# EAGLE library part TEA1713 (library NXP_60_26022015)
Resonant power supply control IC with PFC The TEA1713 integrates a Power Factor Corrector (PFC) controller and a controller for a Half-Bridge resonant Converter (HBC) in a multi-chip IC. It provides the drive function for the discrete MOSFET in an up-converter and for the two discrete power MOSFETs in a resonant half-bridge configuration. The efficient operation of the PFC is achieved by implementing functions such as quasi-resonant operation at high power levels and quasi-resonant operation with valley skipping at lower power levels. OverCurrent Protection (OCP), OverVoltage Protection (OVP), and demagnetization sensing ensure safe operation under all conditions. The HBC module is a is a high-voltage controller for a zero-voltage switching LLC resonant converter. It contains a high-voltage level shift circuit and several protection circuits including OCP, open-loop protection, capacitive mode protection and a general purpose latched protection input. The high-voltage chip is fabricated using a proprietary high-voltage Bipolar-CMOS-DMOS power logic process that enables efficient direct start-up from the rectified universal mains voltage. The low-voltage Silicon On Insulator (SOI) chip is used for accurate, high-speed protection functions and control. The topology of a PFC circuit and a resonant converter controlled by the TEA1713 is very flexible, enabling it to be used in a broad range of applications with a wide mains voltage range. Combining PFC and HBC controllers in a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
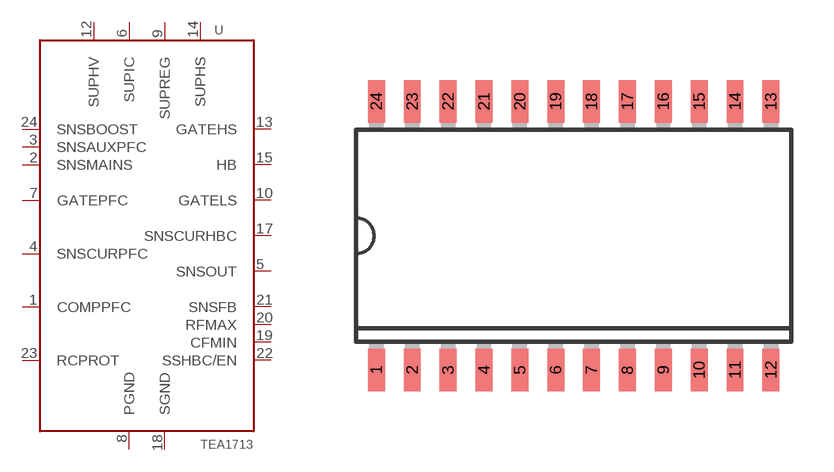
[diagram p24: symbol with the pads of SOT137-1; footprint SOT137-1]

Designator prefix U

## TEA1713T (12NC: 9352 895 98518; FARNELL: 1872212)  [SOT137-1]
1  COMPPFC  pas
2  SNSMAINS  pas
3  SNSAUXPFC  pas
4  SNSCURPFC  pas
5  SNSOUT  out
6  SUPIC  pwr
7  GATEPFC  out
8  PGND  pwr
9  SUPREG  pas
10  GATELS  out
12  SUPHV  in
13  GATEHS  out
14  SUPHS  in
15  HB  in
17  SNSCURHBC  out
18  SGND  pwr
19  CFMIN  pas
20  RFMAX  pas
21  SNSFB  in
22  SSHBC/EN  in
23  RCPROT  pas
24  SNSBOOST  in

## Footprint SOT137-1 (pad centres in mm)
SOT137-1 SO24: plastic small outline package; 24 leads; body width 7.5 mm JEDEC: MS-013 IEC: 075E05
smd 0.6 x 1.5: 1 -6.985,-4.75; 2 -5.715,-4.75; 3 -4.445,-4.75; 4 -3.175,-4.75; 5 -1.905,-4.75; 6 -0.635,-4.75; 7 0.635,-4.75; 8 1.905,-4.75; 9 3.175,-4.75; 10 4.445,-4.75; 11 5.715,-4.75; 12 6.985,-4.75; 13 6.985,4.75; 14 5.715,4.75; 15 4.445,4.75; 16 3.175,4.75; 17 1.905,4.75; 18 0.635,4.75; 19 -0.635,4.75; 20 -1.905,4.75; 21 -3.175,4.75; 22 -4.445,4.75; 23 -5.715,4.75; 24 -6.985,4.75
